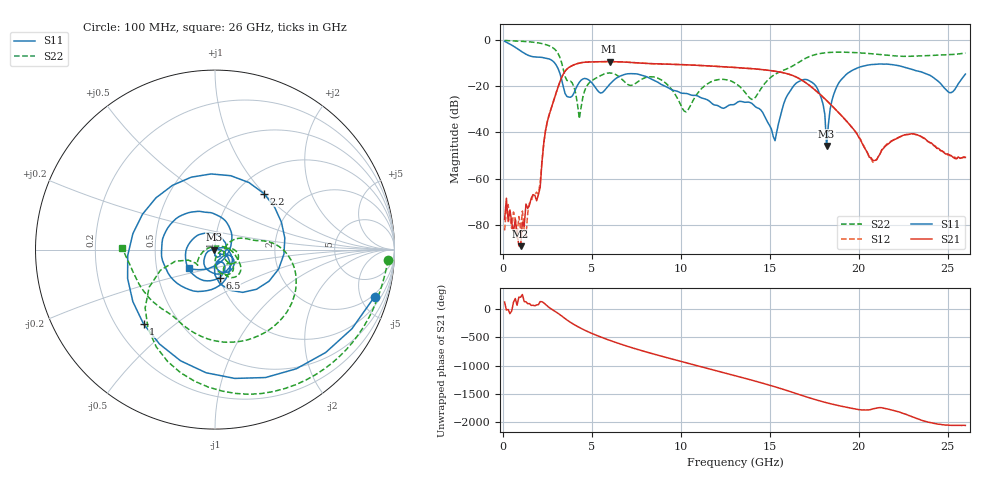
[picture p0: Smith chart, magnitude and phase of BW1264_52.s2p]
!Keysight Technologies,N5245B,MY57181159,A.13.60.06
!Date: Friday, December 18, 2020 23:54:49
!Correction: S11(Full 2 Port(1,2))
!S21(Full 2 Port(1,2))
!S12(Full 2 Port(1,2))
!S22(Full 2 Port(1,2))
!S2P File: Measurements: S11, S21, S12, S22:
# Hz S  dB  R 50
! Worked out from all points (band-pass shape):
!   260 points, 100 MHz to 26 GHz, reference 50 ohm
!   highest |S21| = -9.45 dB at 6 GHz (marker M1); lowest = -89.3 dB at 1 GHz (marker M2)
!   |S21| within 3 dB of the highest: 3.639 GHz to 13.93 GHz (10.29 GHz wide, 117 % of centre)
!   lowest |S11| = -46.0 dB at 18.2 GHz (marker M3), VSWR 1.01, Z = 49.5 + j0.0334 ohm
!   |S11| at or under -10 dB: 2.91 GHz to end of sweep
!   |S22| runs from -34.1 to -0.3 dB; largest |S21 - S12| = 0.00054
!   S11 on the Smith chart (normalised r, x): 100 MHz: 1.74, -6.46; 1 GHz: 0.31, -0.39; 2.2 GHz: 1.32, +1.00; 6.5 GHz: 1.00, -0.32; 26 GHz: 0.73, -0.16
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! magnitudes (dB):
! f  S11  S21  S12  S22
! 100 MHz  -0.7  -77.7  -82.4  -0.3
! 200 MHz  -1.1  -68.5  -73.2  -0.4
! 1 GHz  -4.8  -89.3  -82.1  -0.6
! 1.9 GHz  -7.5  -69.6  -65.9  -1.2
! 2.2 GHz  -7.6  -53.0  -52.6  -1.6
! 3.3 GHz  -17.0  -16.4  -16.4  -9.8
! 4.3 GHz  -18.4  -10.1  -10.1  -34.1
! 4.5 GHz  -17.0  -9.8  -9.8  -24.7
! 6 GHz  -19.3  -9.5  -9.5  -14.4
! 6.5 GHz  -16.0  -9.5  -9.5  -15.8
! 8.8 GHz  -18.8  -10.5  -10.5  -16.9
! 10.3 GHz  -23.2  -10.8  -10.8  -31.2
! 13.1 GHz  -27.5  -12.0  -12.0  -18.9
! 15.3 GHz  -43.6  -13.6  -13.6  -15.0
! 16 GHz  -23.9  -14.7  -14.7  -12.5
! 17.4 GHz  -18.5  -20.8  -20.7  -6.8
! 18 GHz  -27.9  -24.8  -24.8  -5.8
! 18.2 GHz  -46.0  -26.3  -26.2  -5.6
! 18.9 GHz  -18.4  -31.7  -31.8  -5.4
! 20.8 GHz  -10.7  -52.2  -53.0  -6.1
! 21.7 GHz  -10.6  -44.8  -44.6  -6.8
! 26 GHz  -14.8  -50.9  -50.7  -5.7
